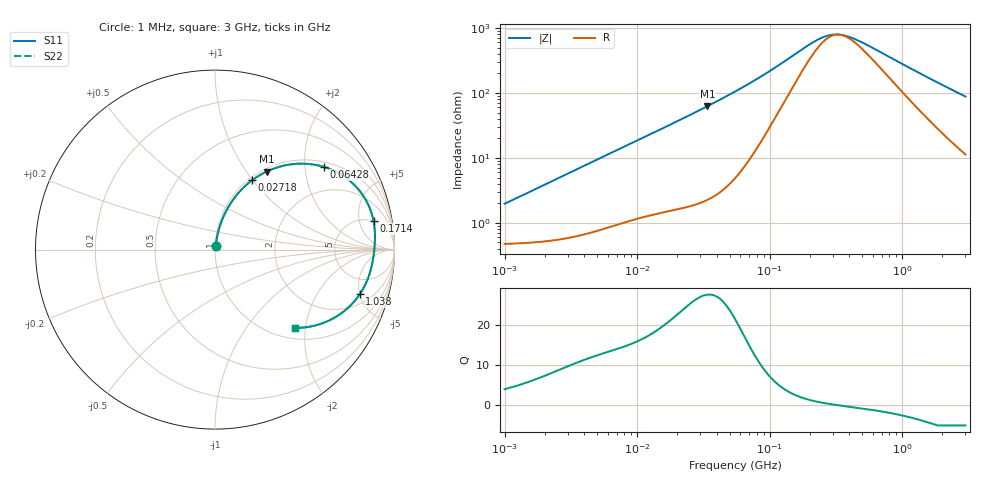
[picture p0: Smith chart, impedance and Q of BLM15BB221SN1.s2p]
! BLM15BB221SN1
# Hz S RI R 50
!Freq.(Hz) S11(Real) S11(Imag) S21(Real) S21(Imag) S12(Real) S12(Imag) S22(Real) S22(Imag)
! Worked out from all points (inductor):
!   401 points, 1 MHz to 3 GHz, reference 50 ohm
!   read as one part in series: L = 305 nH near 1.041 MHz
!   highest Q = 27.6 at 33.88 MHz (marker M1), where L = 294 nH
!   self-resonance near 335.6 MHz
!   S11 on the Smith chart (normalised r, x): 1 MHz: 1.01, +0.04; 27.18 MHz: 1.04, +1.00; 64.28 MHz: 1.15, +2.52; 171.4 MHz: 4.98, +8.17; 1.038 GHz: 2.91, -5.02; 3 GHz: 1.23, -1.75
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1000000  0.00509 0.019  0.9949 -0.019  0.9949 -0.019  0.00509 0.019
3823119  0.0116 0.0713  0.9884 -0.0713  0.9884 -0.0713  0.0116 0.0713
7858845  0.0303 0.1406  0.9697 -0.1406  0.9697 -0.1406  0.0303 0.1406
1.461624e7  0.0781 0.2433  0.9219 -0.2433  0.9219 -0.2433  0.0781 0.2433
2.013356e7  0.1298 0.3147  0.8702 -0.3147  0.8702 -0.3147  0.1298 0.3147
2.718395e7  0.2077 0.3871  0.7923 -0.3871  0.7923 -0.3871  0.2077 0.3871
3.387922e7  0.288 0.4351  0.712 -0.4351  0.712 -0.4351  0.288 0.4351
4.394807e7  0.408 0.4727  0.592 -0.4727  0.592 -0.4727  0.408 0.4727
5.477226e7  0.5235 0.4768  0.4765 -0.4768  0.4765 -0.4768  0.5235 0.4768
6.428402e7  0.6079 0.4601  0.3921 -0.4601  0.3921 -0.4601  0.6079 0.4601
8.338914e7  0.7296 0.3999  0.2704 -0.3999  0.2704 -0.3999  0.7296 0.3999
1.039275e8  0.8057 0.3276  0.1943 -0.3276  0.1943 -0.3276  0.8057 0.3276
1.714156e8  0.8833 0.1593  0.1167 -0.1593  0.1167 -0.1593  0.8833 0.1593
2.094008e8  0.8904 0.1043  0.1096 -0.1043  0.1096 -0.1043  0.8904 0.1043
2.771263e8  0.8907 0.0392  0.1093 -0.0392  0.1093 -0.0392  0.8907 0.0392
3.523638e8  0.8867 -0.00967  0.1133 0.00967  0.1133 0.00967  0.8867 -0.00967
4.66327e8  0.8786 -0.0647  0.1214 0.0647  0.1214 0.0647  0.8786 -0.0647
8.005644e8  0.8431 -0.1826  0.1569 0.1826  0.1569 0.1826  0.8431 -0.1826
1.038491e9  0.807 -0.248  0.193 0.248  0.193 0.248  0.807 -0.248
1.67892e9  0.6847 -0.3678  0.3153 0.3678  0.3153 0.3678  0.6847 -0.3678
2.266846e9  0.5686 -0.4201  0.4314 0.4201  0.4314 0.4201  0.5686 -0.4201
3e9  0.4441 -0.4361  0.5559 0.4361  0.5559 0.4361  0.4441 -0.4361
